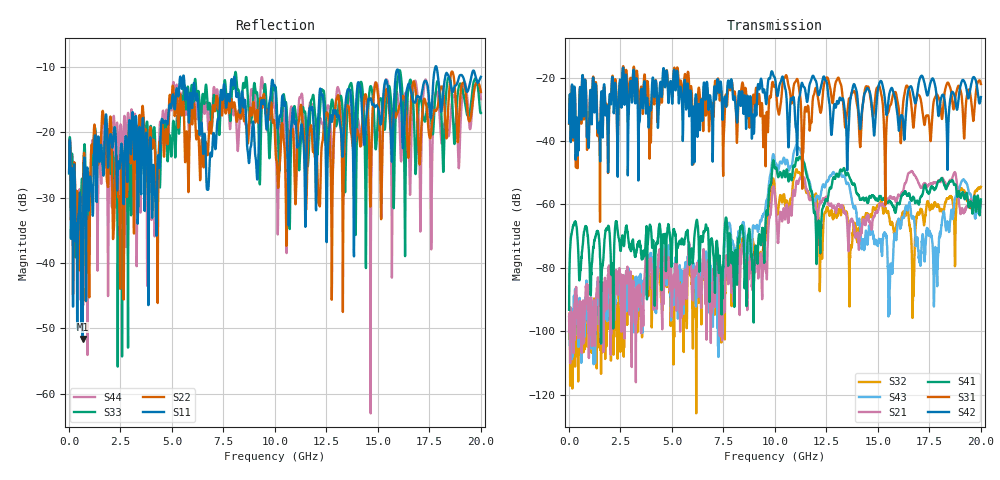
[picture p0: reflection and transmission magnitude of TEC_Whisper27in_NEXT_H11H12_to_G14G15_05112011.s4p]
! Tyco Electronics
! H11H12-G14G15_NEXT
!! PART DESCRIPTION: Whisper 27in Megtron 6 VLP-HVLP-VLP Channel Model, bulkhead 2.4mm test pts
!! MODEL DESCRIPTION: System 4-port S-parameter
!! MODEL STATUS: Measured
!! MODEL GEOMETRY: Channel Model
!! MODEL FREQUENCY RANGE: DC to 20.000 GHz in 10.000 MHz frequency steps
!! MODEL EDGE RATE LIMITATION: 25.00 ps (Using conservative 0.5/Fmax rule of thumb)
!! TIME-DOMAIN TRANSFORM CAUTIONS:
!! 1.) Do not simulate transient edge rates faster than the number listed above.  Edge rates faster than this number
!!  contain significant spectral content at frequencies above the model's highest frequency.
!! 2.) Even when simulating edge rates that are slower than the number listed above, be aware that the best time
!!  resolution possible with a direct iFFT is (1 / 2Fmax).  As a result, time resolution is typically not adequate
!!  for most time-domain simulations unless tricks such as windowing are used to minimize leakage and aliasing.
!! 3.) Because the model has a uniform frequency step, a direct iFFT will result in an impulse that that has a time
!!  length given by either (1 / Fstep) or (1 / 2Fstep), depending on the transform being used.  Care has been taken
!!  in selecting the frequency step to ensure a settled impulse response for the model.  Therefore, convolution with
!!  the model's impulse response should present no issues.  However, if directly concatenating s-parameter models
!!  in the frequency domain a user must either interpolate necessary interim frequencies or complete impulse response
!!  zero-padding.  Impulse response zero-padding is more difficult, but more accurate.
!! PORT DEFINITIONS:
!! Port  1  ----->  Side A  H11  G14  Side A  <-----  Port  2
!! Port  3  ----->  Side A  H12  G15  Side A  <-----  Port  4
! Point-to-Point link (differential)  !
! Connectors:  !
!  1: STRADA Whisper  !
! Materials:  !
!  Backplane: Megtron-6 HVLP  !
!  Daughtercard: Megtron-6 VLP  !
! Stack-up:  !
!  Backplane: 20 layers, 200mil thick  !
!  Daughtercard: 14 layers, 110mil thick  !
! Trace Length:  !
!  Backplane: 17in  !
!  Daightercards: 5in  !
! Trace Width:  !
!  Backplane: 8-13-8 mils  !
!  Daughtercards: 6-9-6 mils  !
! Geometry:  !
!  Backplane: Stripline  !
!  Daughtercards: Stripline  !
! Freq. Range: 0 GHz - 20 GHz  !
! Note1: non-mixed-mode s-parameters  !
! Note2: channel includes 2.4mm test points  !
! Created Wed May 11 15:02:06 2011
! 4 Port Network Data from SP1.SP block
! freq  magS11  angS11  magS12  angS12  magS13  angS13  magS14  angS14
!  magS21  angS21  magS22  angS22  magS23  angS23  magS24  angS24
!  magS31  angS31  magS32  angS32  magS33  angS33  magS34  angS34
!  magS41  angS41  magS42  angS42  magS43  angS43  magS44  angS44
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# hz S ma R 50
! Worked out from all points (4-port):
!   2000 points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, 10 MHz to 20 GHz, reference 50 ohm
!   strongest paths, dB at 10 MHz, 5.01 GHz, 10.01 GHz, 15.01 GHz, 20 GHz:
!     S42: -34.4, -28.0, -20.4, -23.5, -26.1
!     S31: -34.6, -25.5, -22.3, -22.8, -22.0
!     S41: -93.3, -72.9, -48.7, -58.9, -58.4
!     S21: -100.3, -91.1, -57.6, -61.8, -59.1
!     S43: -95.6, -86.8, -46.8, -72.5, -59.3
!     S32: -96.7, -86.2, -56.5, -60.3, -54.4
!   lowest |S11| = -51.6 dB at 670 MHz (marker M1), VSWR 1.01, Z = 49.8 + j0.175 ohm
!   |S11| at or under -10 dB: start of sweep to 17.79 GHz; 17.84 GHz to end of sweep
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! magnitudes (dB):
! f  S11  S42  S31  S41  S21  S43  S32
! 10 MHz  -26.2  -34.4  -34.6  -93.3  -100.3  -95.6  -96.7
! 670 MHz  -51.6  -19.3  -19.3  -72.9  -93.1  -103.0  -104.5
! 8.94 GHz  -18.3  -31.8  -25.8  -82.4  -77.9  -66.7  -71.4
! 11.08 GHz  -22.2  -44.5  -20.4  -45.6  -52.8  -41.7  -49.3
! 12.11 GHz  -17.4  -25.4  -27.3  -65.3  -62.2  -57.9  -63.4
! 15.58 GHz  -16.9  -24.5  -28.9  -59.0  -57.8  -86.3  -65.5
! 20 GHz  -11.5  -26.1  -22.0  -58.4  -59.1  -59.3  -54.4
